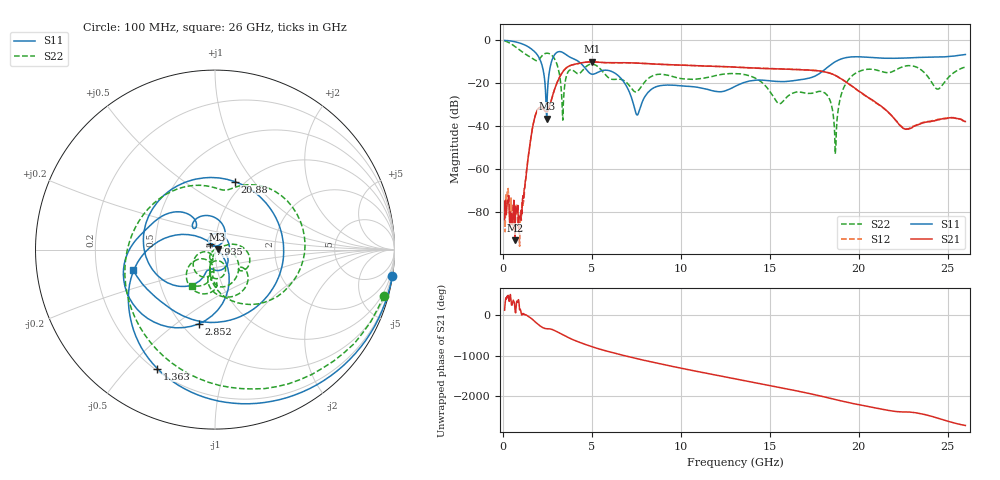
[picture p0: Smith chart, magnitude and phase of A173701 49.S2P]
!  2-Port S-parameters saved by WinCal
! VAR MeasName=S-Parameters (CALIBRATED_DATA) read from VNA (N5245A)
! VAR MeasDate=2017-6-7 10:31:42
! VAR NAME=A173701 49
! VAR FILENAME=A173701 49.S2P
! VAR DATE=2017-6-7 10:31:42
! VAR PHYS_PORTS=1,2
# Hz S DB R 50
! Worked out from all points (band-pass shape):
!   801 points, 100 MHz to 26 GHz, reference 50 ohm
!   highest |S21| = -9.99 dB at 5.021 GHz (marker M1); lowest = -93.4 dB at 682.8 MHz (marker M2)
!   |S21| within 3 dB of the highest: 3.546 GHz to 14.29 GHz (10.75 GHz wide, 121 % of centre)
!   lowest |S11| = -36.5 dB at 2.463 GHz (marker M3), VSWR 1.03, Z = 51.5 + j0.287 ohm
!   |S11| at or under -10 dB: 2.142 GHz to 2.733 GHz (591.7 MHz wide, 24.3 % of centre); 4.28 GHz to 18.67 GHz (14.39 GHz wide, 125 % of centre)
!   |S22| runs from -53.0 to -0.2 dB; largest |S21 - S12| = 0.0034
!   S11 on the Smith chart (normalised r, x): 100 MHz: 0, -13; 1.363 GHz: 0.21, -0.61; 2.852 GHz: 0.60, -0.61; 7.935 GHz: 0.94, +0.06; 20.88 GHz: 0.90, +0.81; 26 GHz: 0.37, -0.11
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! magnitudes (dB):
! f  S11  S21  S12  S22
! 100 MHz  0.0  -83.8  -80.6  -0.2
! 682.8 MHz  -0.6  -93.4  -80.7  -2.8
! 1.071 GHz  -1.6  -81.0  -75.8  -5.2
! 1.363 GHz  -2.7  -59.3  -58.9  -6.9
! 1.848 GHz  -5.8  -34.5  -34.5  -9.4
! 2.463 GHz  -36.5  -33.5  -33.5  -6.0
! 2.852 GHz  -7.5  -24.3  -24.3  -7.9
! 3.37 GHz  -5.7  -14.7  -14.6  -37.2
! 4.438 GHz  -11.2  -10.4  -10.5  -14.4
! 5.021 GHz  -15.8  -10.0  -10.0  -11.1
! 7.935 GHz  -27.0  -10.7  -10.7  -19.9
! 8.744 GHz  -21.3  -11.1  -11.1  -15.8
! 13.05 GHz  -21.5  -12.5  -12.5  -15.5
! 15.51 GHz  -19.2  -13.3  -13.3  -29.5
! 17.39 GHz  -17.2  -14.0  -13.9  -24.7
! 18.26 GHz  -12.5  -15.0  -14.9  -26.0
! 18.68 GHz  -9.9  -16.3  -16.3  -53.0
! 19.36 GHz  -7.9  -19.9  -19.9  -19.1
! 20.88 GHz  -8.1  -28.5  -28.7  -13.6
! 21.69 GHz  -8.4  -33.7  -33.9  -15.1
! 24.45 GHz  -7.7  -37.1  -36.9  -22.7
! 26 GHz  -6.6  -37.9  -37.9  -12.4
